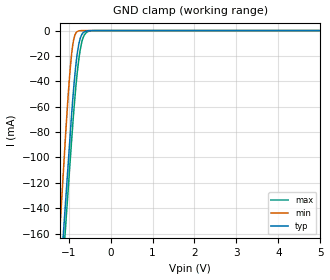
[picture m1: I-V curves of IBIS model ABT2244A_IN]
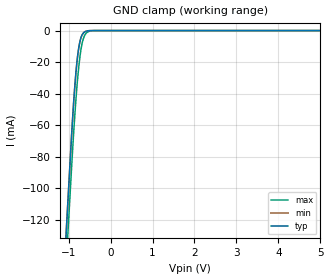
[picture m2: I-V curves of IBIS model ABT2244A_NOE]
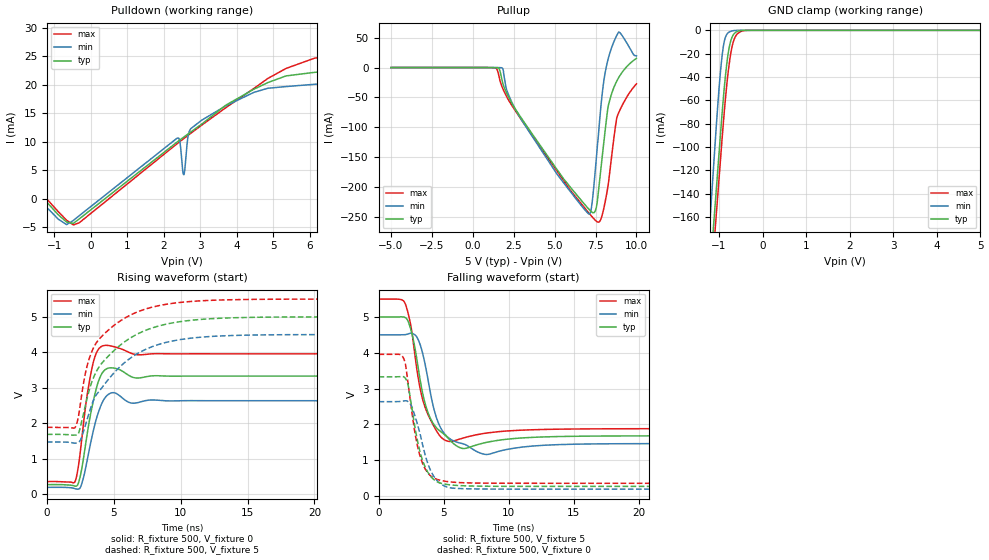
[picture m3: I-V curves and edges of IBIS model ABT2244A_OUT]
| TEXAS INSTRUMENTS INCORPORATED
| Standard Linear and Logic Group
| IBIS Model of SN74ABT2244A
| OCTAL BUFFERS AND LINE/MOS DRIVERS WITH 3-STATE OUTPUTS
| This file contains package information for the following:
|  SOIC 20-pin (DW) package as [Component] ABT2244A_DW
|  SSOP 20-pin (DB) package as [Component] ABT2244A_DB
|  PDIP 20-pin (N) package as [Component] ABT2244A_N
|  TSSOP 20-pin (PW) package as [Component] ABT2244A_PW
| This device can be powered at the following Vccs:
|  5 volt Vcc
| This file provides unique models under the [Model Selector] for each Vcc.
| For operation at a specific Vcc, select the appropriate model after each
| [Model Selector] keyword.
[IBIS Ver]   3.2
[Comment char]  |_char
[File Name]   sn74abt2244a.ibs
[File Rev]   1.2 | j_die
[Date]   September 20, 2006
[Source]   Data created from TI-SPICE simulations at TI-SLL.
[Notes]   The following is an IBIS list for the SN74ABT2244A.
   Please contact sllibis@ti.com with questions and
   comments concerning SLL IBIS models.
   This IBIS model is created from a BA (back annotated netlist)
   - FILE REV HISTORY
   - 1.1 Release IBIS file on 12/17/04
   - 1.2 Release - 9/20/2006 - fixes Pullup waveform issue
   - Non-monotonic data and Decreassing Current warning in pullup
   and pulldown is due to resistor at output.
   - Power clamp data deleted as there is no power-clamp diode.
[Disclaimer] Property of Texas Instruments Incorporated.  Unauthorized
   reproduction and/or distribution is strictly prohibited.
   This product is protected under copyright law.
   Created  2006, (C) Copyright  2006, Texas Instruments
   Incorporated, All Rights Reserved
   UNLESS THERE IS A SIGNED, WRITTEN AGREEMENT TO THE
   CONTRARY, TEXAS INSTRUMENTS (TI) IS PROVIDING THE IBIS
   MODELS  AND WITHOUT ANY WARRANTY, EXPRESSED OR
   IMPLIED.  TI assumes no liability for:
   1) the accuracy of the IBIS models provided to your
   company;
   2) the proper functioning of these IBIS Models in your
   design or for any resulting applications; or
   3) infringement of patents, copyrights or intellectual
   property rights resulting from your use of these IBIS
   models.
   TI provides IBIS Models as a service to our customers.
   You and your company shall not distribute, sell or give
   these models to anyone else without prior written
   permission from TI.
   TI reserves the right to make changes to our products or
   to discontinue any semiconductor product or service
   without notice, and advises our customers to obtain the
   latest version of relevant information to verify, before
   placing orders, that the information being relied on is
   current.
   Please be aware that your receipt and use of the IBIS
   information provided shall serve as acceptance of these
   terms and conditions.  If you do not accept these terms,
   you should return or destroy the IBIS models and any
   other accompanying information immediately.
| Component ABT2244A_DW 20-PIN SOIC
[Component]   ABT2244A_DW
[Manufacturer]   Texas Instruments, Inc.
[Package]
|   typ   min   max
R_pkg   3.800e-02   3.300e-02   4.500e-02
L_pkg   5.012e-09   4.110e-09   6.349e-09
C_pkg   7.170e-13   5.300e-13   8.680e-13
[Pin]   signal_name   model_name   R_pin   L_pin   C_pin
1   1NOE   ABT2244A_NOE   4.200e-02   6.336e-09   8.650e-13
2   1A1   ABT2244A_IN   4.300e-02   5.542e-09   8.670e-13
3   2Y4   ABT2244A_OUT   3.400e-02   4.714e-09   7.320e-13
4   1A2   ABT2244A_IN   3.400e-02   4.377e-09   5.910e-13
5   2Y3   ABT2244A_OUT   3.600e-02   4.130e-09   5.330e-13
6   1A3   ABT2244A_IN   3.500e-02   4.111e-09   5.300e-13
7   2Y2   ABT2244A_OUT   3.400e-02   4.284e-09   5.830e-13
8   1A4   ABT2244A_IN   3.400e-02   4.634e-09   7.260e-13
9   2Y1   ABT2244A_OUT   4.000e-02   5.518e-09   8.650e-13
10   GND   GND   4.300e-02   6.349e-09   8.660e-13
11   2A1   ABT2244A_IN   4.100e-02   6.281e-09   8.610e-13
12   1Y4   ABT2244A_OUT   4.500e-02   5.561e-09   8.680e-13
13   2A2   ABT2244A_IN   3.300e-02   4.778e-09   7.420e-13
14   1Y3   ABT2244A_OUT   3.500e-02   4.414e-09   5.960e-13
15   2A3   ABT2244A_IN   3.500e-02   4.110e-09   5.330e-13
16   1Y2   ABT2244A_OUT   3.600e-02   4.130e-09   5.330e-13
17   2A4   ABT2244A_IN   3.400e-02   4.377e-09   5.910e-13
18   1Y1   ABT2244A_OUT   3.400e-02   4.714e-09   7.310e-13
19   2NOE   ABT2244A_NOE   4.300e-02   5.569e-09   8.680e-13
20   VCC   POWER   4.200e-02   6.308e-09   8.640e-13
| Component ABT2244A_DB 20-PIN SSOP
[Component]   ABT2244A_DB
[Manufacturer]   Texas Instruments, Inc.
[Package]
|   typ   min   max
R_pkg   4.000e-02   3.500e-02   5.100e-02
L_pkg   3.495e-09   3.035e-09   4.314e-09
C_pkg   4.200e-13   3.460e-13   5.020e-13
[Pin]   signal_name   model_name   R_pin   L_pin   C_pin
1   1NOE   ABT2244A_NOE   4.900e-02   4.310e-09   5.020e-13
2   1A1   ABT2244A_IN   4.800e-02   3.903e-09   4.870e-13
3   2Y4   ABT2244A_OUT   3.500e-02   3.189e-09   3.960e-13
4   1A2   ABT2244A_IN   3.500e-02   3.036e-09   3.470e-13
5   2Y3   ABT2244A_OUT   3.500e-02   3.035e-09   3.670e-13
6   1A3   ABT2244A_IN   3.500e-02   3.035e-09   3.670e-13
7   2Y2   ABT2244A_OUT   3.500e-02   3.036e-09   3.470e-13
8   1A4   ABT2244A_IN   3.500e-02   3.189e-09   3.970e-13
9   2Y1   ABT2244A_OUT   4.700e-02   3.899e-09   4.880e-13
10   GND   GND   5.100e-02   4.314e-09   5.000e-13
11   2A1   ABT2244A_IN   5.100e-02   4.314e-09   5.000e-13
12   1Y4   ABT2244A_OUT   4.700e-02   3.899e-09   4.880e-13
13   2A2   ABT2244A_IN   3.500e-02   3.189e-09   3.970e-13
14   1Y3   ABT2244A_OUT   3.500e-02   3.036e-09   3.460e-13
15   2A3   ABT2244A_IN   3.500e-02   3.035e-09   3.670e-13
16   1Y2   ABT2244A_OUT   3.500e-02   3.035e-09   3.670e-13
17   2A4   ABT2244A_IN   3.500e-02   3.036e-09   3.460e-13
18   1Y1   ABT2244A_OUT   3.500e-02   3.189e-09   3.970e-13
19   2NOE   ABT2244A_NOE   4.700e-02   3.899e-09   4.880e-13
20   VCC   POWER   5.100e-02   4.314e-09   5.020e-13
| Component ABT2244A_N 20-PIN PDIP
[Component]   ABT2244A_N
[Manufacturer]   Texas Instruments, Inc.
[Package]
|   typ   min   max
R_pkg   4.300e-02   3.800e-02   5.000e-02
L_pkg   7.384e-09   4.680e-09   1.032e-08
C_pkg   5.100e-13   2.310e-13   8.210e-13
[Pin]   signal_name   model_name   R_pin   L_pin   C_pin
1   1NOE   ABT2244A_NOE   4.200e-02   9.427e-09   8.100e-13
2   1A1   ABT2244A_IN   4.600e-02   8.544e-09   4.560e-13
3   2Y4   ABT2244A_OUT   4.800e-02   7.163e-09   4.350e-13
4   1A2   ABT2244A_IN   4.000e-02   4.825e-09   2.610e-13
5   2Y3   ABT2244A_OUT   4.000e-02   5.284e-09   6.480e-13
6   1A3   ABT2244A_IN   4.000e-02   4.686e-09   2.320e-13
7   2Y2   ABT2244A_OUT   4.000e-02   6.359e-09   4.890e-13
8   1A4   ABT2244A_IN   3.800e-02   7.982e-09   4.750e-13
9   2Y1   ABT2244A_OUT   4.300e-02   9.403e-09   4.750e-13
10   GND   GND   5.000e-02   1.032e-08   8.050e-13
11   2A1   ABT2244A_IN   5.000e-02   1.028e-08   8.100e-13
12   1Y4   ABT2244A_OUT   4.300e-02   9.383e-09   4.770e-13
13   2A2   ABT2244A_IN   3.800e-02   7.978e-09   4.760e-13
14   1Y3   ABT2244A_OUT   4.000e-02   6.302e-09   4.920e-13
15   2A3   ABT2244A_IN   4.000e-02   4.680e-09   2.310e-13
16   1Y2   ABT2244A_OUT   4.000e-02   5.284e-09   6.480e-13
17   2A4   ABT2244A_IN   4.000e-02   4.822e-09   2.610e-13
18   1Y1   ABT2244A_OUT   4.700e-02   7.118e-09   4.390e-13
19   2NOE   ABT2244A_NOE   4.600e-02   8.492e-09   4.610e-13
20   VCC   POWER   4.300e-02   9.348e-09   8.210e-13
| Component ABT2244A_PW 20-PIN TSSOP
[Component]   ABT2244A_PW
[Manufacturer]   Texas Instruments, Inc.
[Package]
|   typ   min   max
R_pkg   5.000e-02   4.200e-02   6.000e-02
L_pkg   2.802e-09   2.248e-09   3.553e-09
C_pkg   3.170e-13   2.020e-13   4.430e-13
[Pin]   signal_name   model_name   R_pin   L_pin   C_pin
1   1NOE   ABT2244A_NOE   5.500e-02   3.461e-09   4.400e-13
2   1A1   ABT2244A_IN   5.500e-02   3.150e-09   4.010e-13
3   2Y4   ABT2244A_OUT   4.200e-02   2.619e-09   3.020e-13
4   1A2   ABT2244A_IN   4.500e-02   2.273e-09   2.020e-13
5   2Y3   ABT2244A_OUT   4.500e-02   2.248e-09   2.240e-13
6   1A3   ABT2244A_IN   4.500e-02   2.273e-09   2.260e-13
7   2Y2   ABT2244A_OUT   4.400e-02   2.323e-09   2.050e-13
8   1A4   ABT2244A_IN   4.600e-02   2.704e-09   3.070e-13
9   2Y1   ABT2244A_OUT   6.000e-02   3.265e-09   4.110e-13
10   GND   GND   5.700e-02   3.506e-09   4.360e-13
11   2A1   ABT2244A_IN   5.800e-02   3.553e-09   4.370e-13
12   1Y4   ABT2244A_OUT   5.800e-02   3.193e-09   4.050e-13
13   2A2   ABT2244A_IN   4.200e-02   2.704e-09   3.110e-13
14   1Y3   ABT2244A_OUT   4.600e-02   2.392e-09   2.100e-13
15   2A3   ABT2244A_IN   4.700e-02   2.334e-09   2.290e-13
16   1Y2   ABT2244A_OUT   4.700e-02   2.300e-09   2.270e-13
17   2A4   ABT2244A_IN   4.700e-02   2.349e-09   2.070e-13
18   1Y1   ABT2244A_OUT   4.500e-02   2.677e-09   3.060e-13
19   2NOE   ABT2244A_NOE   6.000e-02   3.235e-09   4.060e-13
20   VCC   POWER   5.600e-02   3.487e-09   4.430e-13
| Models and submodels in the file (3): ABT2244A_IN (Input), ABT2244A_NOE (Input), ABT2244A_OUT (3-state)
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[Model]   ABT2244A_IN
Model_type  Input
Vinl=0.8
Vinh=2.0
| variable   typ   min   max
C_comp   2.97pF   2.25pF   4.48pF
[Temperature Range]   40   -40   100
| Ambient temperature   25   -40   85
[Voltage range]   5   4.5   5.5
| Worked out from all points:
|   GND clamp passes 1 mA (typ) near -0.62 V on its own axis
[GND Clamp]
| ABT2244A_IN
|   Voltage   I(typ)   I(min)   I(max)
-5V       -2.023A    -2.247A    -2.022A
-1.87V    -519.1mA   -522.7mA   -534.7mA
-1.075V   -137mA     -84.7mA    -156.8mA
-1V       -100.9mA   -46.9mA    -121.2mA
-925mV    -65.25mA   -17.85mA   -85.55mA
-900mV    -54.4mA    -11.35mA   -74.27mA
-850mV    -35.11mA   -3.716mA   -53.41mA
-775mV    -14.29mA   -457.6uA   -27.94mA
-725mV    -6.493mA   -67.43uA   -15.76mA
-650mV    -1.652mA   -2.017uA   -5.335mA
-475mV    -17.97uA   -673.5pA   -221.3uA
5V        34.17pA    24.48pA    478.5pA
[Model]   ABT2244A_NOE
Model_type  Input
Vinl=0.8
Vinh=2.0
| variable   typ   min   max
C_comp   2.90pF   2.22pF   4.34pF
[Temperature Range]   40   -40   100
| Ambient temperature   25   -40   85
[Voltage range]   5   4.5   5.5
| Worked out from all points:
|   GND clamp passes 1 mA (typ) near -0.62 V on its own axis
[GND Clamp]
| ABT2244A_NOE
|   Voltage   I(typ)   I(min)   I(max)
-5V       -2.023A    -2.023A    -2.022A
-1.545V   -362.9mA   -362.9mA   -380.2mA
-950mV    -76.91mA   -76.9mA    -97.43mA
-900mV    -54.4mA    -54.38mA   -74.27mA
-850mV    -35.11mA   -35.1mA    -53.41mA
-800mV    -19.82mA   -19.8mA    -35.31mA
-775mV    -14.29mA   -14.27mA   -27.94mA
-700mV    -4.17mA    -4.158mA   -11.25mA
-650mV    -1.652mA   -1.644mA   -5.335mA
-600mV    -594.3uA   -589.7uA   -2.353mA
-375mV    -575.3nA   -570.4nA   -15.8uA
5V        34.17pA    37.42pA    478.5pA
[Model]   ABT2244A_OUT
Model_type  3-state
Enable   Active-Low
Vref =   0
Rref =   500
Cref =   50p
Vmeas =   1.5
| variable   typ   min   max
C_comp   5.64pF   4.18pF   8.52pF
| C_pullup   5.88pF   4.22pF   8.77pF
| C_pulldown   6.64pF   5.55pF   7.81pF
| C_tri-state   5.64pF   4.18pF   8.52pF
[Temperature Range]   40   -40   100
| Ambient temperature   25   -40   85
[Voltage range]   5   4.5   5.5
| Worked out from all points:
|   slope of the pulldown table from 0 to 0.75 V, typ, clamps not added: 199 ohm
|   GND clamp passes 1 mA (typ) near -0.58 V on its own axis
|   rising waveform, R_fixture 500, V_fixture 0: 20-80 % time 846ps typ, 852ps min, 748ps max; typ from 0.265 V to 3.33 V
|   falling waveform, R_fixture 500, V_fixture 5: 20-80 % time 1.09ns typ, 1.11ns min, 992ps max; typ from 5 V to 1.68 V
|   rising waveform, R_fixture 500, V_fixture 5: 20-80 % time 3.19ns typ, 3.49ns min, 2.56ns max; typ from 1.68 V to 5 V
|   falling waveform, R_fixture 500, V_fixture 0: 20-80 % time 1.05ns typ, 1.17ns min, 989ps max; typ from 3.33 V to 0.265 V
[GND Clamp]
| ABT2244A_OUT
|   Voltage   I(typ)   I(min)   I(max)
-5V       -2.331A    -2.66A     -2.351A
-1.335V   -271mA     -235.5mA   -291mA
-1.075V   -142.9mA   -89.12mA   -164.1mA
-1V       -105.9mA   -50.47mA   -127.5mA
-925mV    -69.35mA   -20.59mA   -90.96mA
-875mV    -47.7mA    -8.852mA   -68.17mA
-825mV    -29.82mA   -3.629mA   -48.11mA
-750mV    -11.95mA   -1.123mA   -24.62mA
-700mV    -5.789mA   -520.9uA   -13.97mA
-625mV    -1.917mA   -77.31uA   -5.43mA
-400mV    -5.677uA   -2.715nA   -135.7uA
5V        443.2pA    566.9pA    3.942nA
[Pulldown]
| ABT2244A_OUT
|   Voltage   I(typ)   I(min)   I(max)
-5V       87.03mA    151.7mA    69.44mA
-2.765V   58.19mA    30.42mA    85.56mA
-2.65V    38.5mA     12.91mA    66.52mA
-2.425V   12.09mA    7.989mA    31.15mA
-2.24V    7.076mA    6.411mA    12.02mA
-2.045V   5.328mA    4.908mA    5.869mA
-475mV    -4.319mA   -3.806mA   -4.59mA
2.37V     9.953mA    10.64mA    9.664mA
2.55V     10.8mA     4.205mA    10.54mA
2.74V     11.69mA    12.27mA    11.46mA
4.465V    19.18mA    18.63mA    19.31mA
10V       24.13mA    21.89mA    27.03mA
[Pullup]
| ABT2244A_OUT
|   Voltage   I(typ)   I(min)   I(max)
-5V       -35.32pA   -25.92pA   -27.91pA
1.355V    -85.12uA   -693.5nA   -421.2uA
1.805V    -23.08mA   -738.6uA   -33.02mA
2.08V     -42.99mA   -37.95mA   -49.08mA
2.74V     -75.18mA   -76.75mA   -77.99mA
7.115V    -237.5mA   -245mA     -244mA
7.29V     -242.1mA   -226.1mA   -249.6mA
7.57V     -231.1mA   -145mA     -257.5mA
7.965V    -135mA     -30.59mA   -240.3mA
8.36V     -55.31mA   23.1mA     -177mA
8.815V    -21.69mA   54.73mA    -82.39mA
10V       15.42mA    19.49mA    -27.18mA
[Ramp]
| ABT2244A_OUT
| variable   typ   min   max
dV/dt_r   2.00/9.52E-10   1.63/9.95E-10   2.33/8.32E-10
dV/dt_f   2.21/1.41E-09   2.04/1.41E-09   2.39/1.24E-09
R_load = 500
[Rising Waveform]
| ABT2244A_OUT
R_fixture =   500
C_fixture =   0
L_fixture =   0
V_fixture =   0
V_fixture_min = 0
V_fixture_max = 0
|   Time   V(typ)   V(min)   V(max)
0s        265.5mV    187.8mV    352.3mV
2.12ns    222mV      147.3mV    364mV
2.58ns    658.5mV    259.4mV    1.462V
2.955ns   1.552V     843.7mV    2.65V
3.36ns    2.427V     1.599V     3.536V
3.745ns   3.047V     2.18V      4.017V
4.26ns    3.474V     2.666V     4.189V
4.985ns   3.555V     2.86V      4.159V
6.9ns     3.274V     2.589V     3.927V
50ns      3.327V     2.633V     3.955V
[Falling Waveform]
| ABT2244A_OUT
R_fixture =   500
C_fixture =   0
L_fixture =   0
V_fixture =   5
V_fixture_min = 4.5
V_fixture_max = 5.5
|   Time   V(typ)   V(min)   V(max)
0s        5V         4.5V       5.5V
1.995ns   4.992V     4.505V     5.409V
2.46ns    4.669V     4.548V     4.788V
2.92ns    3.862V     4.45V      3.587V
3.835ns   2.289V     3.17V      2.241V
4.49ns    1.887V     2.138V     1.793V
5.33ns    1.616V     1.636V     1.527V
6.47ns    1.325V     1.458V     1.614V
8.28ns    1.495V     1.157V     1.755V
50ns      1.683V     1.466V     1.881V
[Rising Waveform]
| ABT2244A_OUT
R_fixture =   500
C_fixture =   0
L_fixture =   0
V_fixture =   5
V_fixture_min = 4.5
V_fixture_max = 5.5
|   Time   V(typ)   V(min)   V(max)
0s        1.683V     1.467V     1.881V
2.13ns    1.663V     1.435V     1.891V
2.415ns   1.768V     1.475V     2.318V
3.05ns    2.767V     2.154V     3.676V
3.535ns   3.327V     2.691V     4.164V
4ns       3.638V     2.944V     4.408V
6.085ns   4.365V     3.79V      5.018V
8.55ns    4.759V     4.241V     5.328V
15.39ns   4.984V     4.485V     5.49V
50ns      5V         4.5V       5.5V
[Falling Waveform]
| ABT2244A_OUT
R_fixture =   500
C_fixture =   0
L_fixture =   0
V_fixture =   0
V_fixture_min = 0
V_fixture_max = 0
|   Time   V(typ)   V(min)   V(max)
0s        3.327V     2.633V     3.955V
1.91ns    3.332V     2.652V     3.853V
2.08ns    3.273V     2.659V     3.641V
2.275ns   3.084V     2.631V     3.111V
2.79ns    1.929V     2.232V     1.772V
3.235ns   1.163V     1.657V     1.055V
3.985ns   554.4mV    719.4mV    563.8mV
4.925ns   340.5mV    302.5mV    421.1mV
8.125ns   270.2mV    191.4mV    355.9mV
50ns      265.4mV    187.9mV    352.4mV
